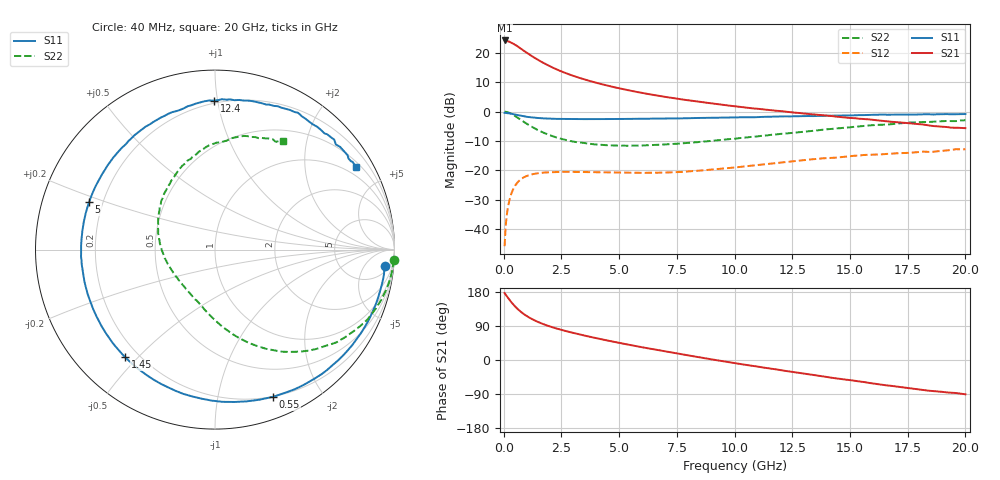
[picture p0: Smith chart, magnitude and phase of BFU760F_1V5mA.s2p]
! Filename:  P:\Prog\Test\Noise\ATS_data\Testdata_Net\Split files Spar\BFU760_2W_C1_1V_5mA_60mA_Bias1_D.s2p
! Date/Time: Mon 06/Feb/2012 15:05:57
! BFU760_2W_C1_1V_5mA_60mA_Bias1_R.s2p
! MDIF S-parameter v. bias file
! BFU760_2W_C1_1V_5mA_60mA
! Date/time Fri Mar 18 10:56:44 2011
! bias mode 1
! bias variable = I_out
! VAR bias_var= 1
! VAR V_out= 1.0002
! VAR I_out= 5.0050
! VAR V_in= 0.7584
! VAR I_in= 0.0139
! Device data file deembeded for feedlines and parallel
! Original file: \Split files Spar\BFU760_2W_C1_1V_5mA_60mA_Bias1_R.s2p
! Feed-files: PR003V01_101208_Feed1.s2p, PR003V01_101208_Feed2.s2p
! Parallel-file: PR003V01_101208_Par.s2p
# MHz S MA R 50
!  Freq-MHz  S11-mag  S11-arg  S21-mag  S21-arg  S12-mag  S12-arg  S22-mag  S22-arg
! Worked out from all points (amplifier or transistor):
!   167 points, 40 MHz to 20 GHz, reference 50 ohm
!   highest |S21| = 24.2 dB at 50 MHz (marker M1)
!   |S21| within 3 dB of that: start of sweep to 786.3 MHz
!   unconditionally stable (mu >= 1): 6.065 GHz to 13.76 GHz
!   at 550 MHz: K = 0.07, MSG = 23.5 dB, |S12| = -24.6 dB
!   at 4.2 GHz: K = 0.68, MSG = 15.0 dB, |S12| = -20.6 dB
!   at 20 GHz: K = 0.83, MSG = 3.6 dB, |S12| = -12.8 dB
!   S11 on the Smith chart (normalised r, x): 40 MHz: 9, -17; 550 MHz: 0.20, -1.45; 1.45 GHz: 0.15, -0.46; 5 GHz: 0.15, +0.18; 12.4 GHz: 0.18, +0.98; 20 GHz: 0.67, +3.57
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40  0.952 -5.5  16.18 176.7  0.005162 86.9  0.9971 -3.4
50  0.9492 -6.9  16.2 175.3  0.00625 82.9  0.9963 -4.3
60  0.9515 -8.1  15.98 174.6  0.007593 86.2  0.996 -5.0
80  0.9505 -10.9  16.12 173.0  0.01036 84.3  0.9937 -6.7
140  0.9463 -19.0  15.9 167.8  0.01809 79.8  0.9837 -11.8
280  0.9284 -37.3  15.18 156.3  0.03479 69.8  0.9408 -23.0
420  0.9041 -54.4  14.29 146.1  0.04886 60.6  0.8791 -33.1
550  0.8819 -68.4  13.27 137.8  0.05919 53.1  0.8132 -41.5
750  0.8492 -87.1  11.74 126.9  0.07107 43.8  0.7209 -52.2
1000  0.8168 -105.7  10.01 116.0  0.0806 34.8  0.6221 -62.7
1250  0.7933 -120.3  8.62 107.3  0.08634 28.2  0.5432 -71.1
1450  0.7812 -129.9  7.728 101.4  0.08919 24.0  0.4922 -76.8
1800  0.7653 -143.1  6.474 92.8  0.0924 18.3  0.426 -85.2
2200  0.7547 -154.7  5.424 84.7  0.09396 13.6  0.3725 -93.3
3400  0.7459 -178.7  3.621 65.9  0.09428 4.9  0.2954 -113.3
5000  0.7497 159.3  2.491 45.2  0.09185 0.4  0.2633 -137.4
6800  0.7616 139.9  1.834 24.8  0.09174 0.3  0.2741 -162.2
10200  0.8002 108.9  1.209 -10.1  0.1143 1.1  0.3543 153.6
12400  0.8303 90.4  0.9833 -30.5  0.1418 -4.8  0.4311 128.6
13400  0.8394 82.5  0.8986 -39.3  0.1553 -10.1  0.4714 118.0
16800  0.8863 55.4  0.6709 -68.3  0.1926 -29.6  0.6111 83.7
20000  0.9095 30.3  0.5237 -90.5  0.2291 -51.6  0.7136 57.9
